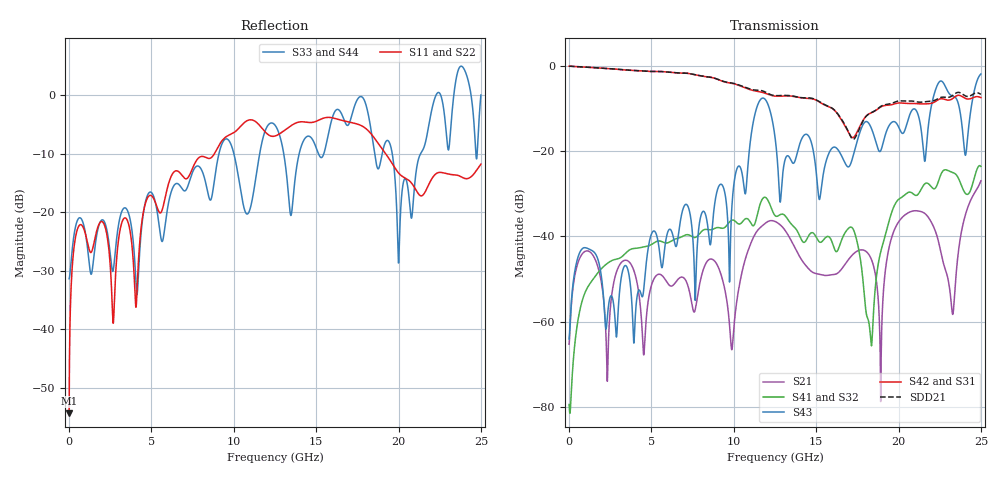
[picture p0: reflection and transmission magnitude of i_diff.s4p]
!Keysight Technologies,N5245B,MY57181346,A.12.70.07
!Automatic Fixture Removal (AFR)
!Date: Wednesday, November 07, 2018 11:53:10 AM
!S4P File: Measurements: <S11,S12,S13,S14>,
!<S21,S22,S23,S24>,
!<S31,S32,S33,S34>,
!<S41,S42,S43,S44>:
# MHz S  RI  R 50
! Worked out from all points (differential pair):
!   2499 points, 10 MHz to 24.99 GHz, reference 50 ohm
!   strongest paths, dB at 10 MHz, 6.25 GHz, 12.5 GHz, 18.75 GHz, 24.99 GHz:
!     S42: 0.0, -1.5, -7.0, -10.0, -7.4
!     S31: 0.0, -1.5, -7.0, -10.0, -7.4
!     S43: -64.1, -39.0, -16.7, -19.5, -1.8
!     S41: -79.5, -41.0, -35.1, -46.8, -23.6
!     S32: -79.5, -41.0, -35.1, -46.8, -23.6
!     S21: -65.3, -51.6, -36.5, -54.2, -26.9
!   taken as a pair (ports 2,1 in; 4,3 out), SDD21 dB: 0.0, -1.5, -6.9, -9.9, -6.6
!   lowest |S11| = -54.3 dB at 10 MHz (marker M1), VSWR 1.00, Z = 50.1 + j0.177 ohm
!   |S11| at or under -10 dB: start of sweep to 8.831 GHz; 19.2 GHz to end of sweep
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10  0.000773 0.00177  0.000534 8.93e-05  0.9996 -0.0202  0.000106 7.63e-06
    0.000534 8.93e-05  0.000773 0.00177  0.000106 7.63e-06  0.9996 -0.0202
    0.9996 -0.0202  0.000106 7.63e-06  0.027 0.00151  -0.000614 0.000119
    0.000106 7.63e-06  0.9996 -0.0202  -0.000614 0.000119  0.027 0.00151
1540  -0.0555 0.0109  -0.00427 -0.00367  -0.9589 -0.0386  0.000608 -0.00324
      -0.00427 -0.00367  -0.0555 0.0109  0.000608 -0.00324  -0.9589 -0.0386
      -0.9589 -0.0386  0.000608 -0.00324  0.0434 0.0141  0.00546 -0.00352
      0.000608 -0.00324  -0.9589 -0.0386  0.00546 -0.00352  0.0434 0.0141
3100  -0.0537 0.0458  -0.00467 0.000681  0.9112 0.0536  -0.000523 0.00556
      -0.00467 0.000681  -0.0537 0.0458  -0.000523 0.00556  0.9112 0.0536
      0.9112 0.0536  -0.000523 0.00556  0.0443 0.0791  0.0015 0.00208
      -0.000523 0.00556  0.9112 0.0536  0.0015 0.00208  0.0443 0.0791
4690  -0.121 0.033  -0.000922 0.000579  -0.8709 -0.0343  0.000844 -0.00758
      -0.000922 0.000579  -0.121 0.033  0.000844 -0.00758  -0.8709 -0.0343
      -0.8709 -0.0343  0.000844 -0.00758  0.1244 0.0378  -0.00102 0.00476
      0.000844 -0.00758  -0.8709 -0.0343  -0.00102 0.00476  0.1244 0.0378
21910  -0.0555 -0.1728  -0.00515 -0.0147  0.1743 0.3191  0.018 -0.0355
       -0.00515 -0.0147  -0.0555 -0.1728  0.018 -0.0355  0.1743 0.3191
       0.1743 0.3191  0.018 -0.0355  0.517 -0.3675  0.1242 -0.2539
       0.018 -0.0355  0.1743 0.3191  0.1242 -0.2539  0.517 -0.3675
23600  -0.0508 -0.1994  0.00575 -0.00173  -0.3495 -0.2907  0.0069 0.0489
       0.00575 -0.00173  -0.0508 -0.1994  0.0069 0.0489  -0.3495 -0.2907
       -0.3495 -0.2907  0.0069 0.0489  -1.568 0.3094  0.3659 -0.0801
       0.0069 0.0489  -0.3495 -0.2907  0.3659 -0.0801  -1.568 0.3094
24990  -0.0175 -0.2559  -0.0135 -0.0429  0.1472 0.4015  -0.0652 -0.0127
       -0.0135 -0.0429  -0.0175 -0.2559  -0.0652 -0.0127  0.1472 0.4015
       0.1472 0.4015  -0.0652 -0.0127  0.9157 0.3939  0.00156 -0.8094
       -0.0652 -0.0127  0.1472 0.4015  0.00156 -0.8094  0.9157 0.3939
